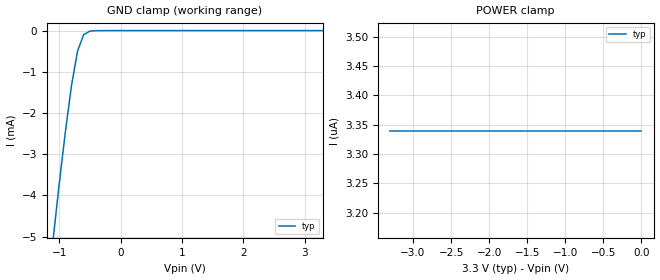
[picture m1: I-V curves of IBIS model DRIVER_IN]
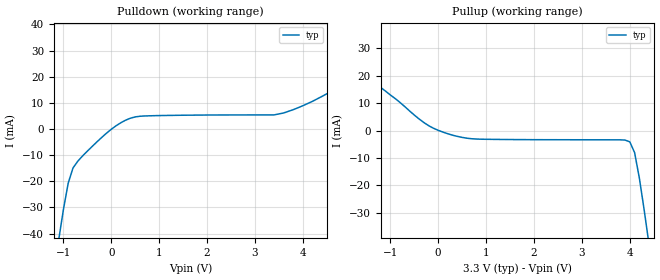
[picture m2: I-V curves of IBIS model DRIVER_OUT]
|   Texas Instruments Incorporated
|   Data Transmissions Products
|   IBIS Model for SN65LVDS1
|   5DBV SOP Package
[IBIS Ver]   2.1
[Comment char]   |_char
[File name]   lvds1.ibs
[File Rev]   1.0
[Date]   11Jan00
[Source]   File originated at Texas Instruments Incorporated.
   Data Transmission Products Group.
[Notes]
[Disclaimer]
(C) Copyright Texas Instruments Incorporated 2000
   All rights reserved
  Texas Instruments Incorporated hereby grants the user of this IBIS
model a non-exclusive, nontransferable license to use this IBIS model
under the following terms.  Before using this IBIS model, the user
should read this license.  If the user does not accept these terms,
the IBIS model should be returned to Texas Instruments within 30 days.
  The user is granted this license only to use the IBIS model and
is not granted rights to sell, load, rent, lease or license the IBIS
model in whole or in part, or in modified form to anyone other than
user.  User may modify the IBIS model to suit its specific applications
but rights to derivative works and such modifications shall belong to
Texas Instruments.
  This IBIS model is provided on an "AS IS" basis and Texas Instruments
makes absolutely no warranty with respect to the information contained
herein.  TEXAS INSTRUMENTS DISCLAIMS AND CUSTOMER WAIVES ALL WARRANTIES,
EXPRESS OR IMPLIED, INCLUDING WARRANTIES OF MERCHANTABILITY OR FITNESS
FOR A PARTICULAR PURPOSE. The entire risk as to quality and performance
is with the Customer. ACCORDINGLY, IN NO EVENT SHALL THE COMPANY BE LIABLE
FOR ANY DAMAGES, WHETHER IN CONTRACT OR TORT,INCLUDING ANY LOST PROFITS
OR OTHER INCIDENTAL, CONSEQUENTIAL, EXEMPLARY, OR PUNITIVE DAMAGES ARISING
OUT OF THE USE OR APPLICATION OF THE IBIS model provided in this package.
Further, Texas Instruments reserves the right to discontinue or make changes
without notice to any product herein to improve reliability, function, or
design. Texas Instruments does not convey any license under patent rights
or any other intellectual property rights, including those of third parties.
Contact Texas Instruments at ATTN:DATA TRANSMISSIONS
[Copyright]   Copyright 2000, Texas Instruments, All Rights Reserved
[Component]   LVDS1DBV
[Manufacturer]  Texas Instruments Incorporated
[Package]
|   typ   min   max
R_pkg   0.036   0.033   0.039
L_pkg   3.340nH   2.445nH   4.233nH
C_pkg   0.470pF   0.308pF   0.631pF
[Pin]   signal_name   model_name   R_pin   L_pin   C_pin
1   VCC   POWER   0.034   4.233n   0.630p
2   GND   GND   0.033   4.231n   0.631p
3   Z   DRIVER_OUT   0.033   4.230n   0.630p
4   Y   DRIVER_OUT   0.033   4.230n   0.630p
5   D   DRIVER_IN   0.033   4.230n   0.630p
[Diff_pin]   inv_pin   vdiff   tdelay_typ   tdelay_min   tdelay_max
| The 'Z' pin is Diff_pin and the 'Y' pin is the inv_pin
4   3   0.100   0 0 0
| Models and submodels in the file (2): DRIVER_IN (Input), DRIVER_OUT (Output)
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|   Driver Input MODEL
[Model]   DRIVER_IN
Model_type   Input
|Signals   D
Vinh = 2.0
Vinl = 0.8
|   typ   min   max
C_comp   1.0pF   NA   NA
|   typ   min   max
[Temperature Range]   25.0   NA   NA
[Voltage range]   3.3V   3.0V   3.6V
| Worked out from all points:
|   GND clamp passes 1 mA (typ) near -0.76 V on its own axis
[GND_clamp]
|   Voltage   I(typ)   I(min)   I(max)
-3.3V     -43.1mA    NA         NA
-1.1V     -5.08mA    NA         NA
-1V       -3.73mA    NA         NA
-900mV    -2.47mA    NA         NA
-800mV    -1.34mA    NA         NA
-700mV    -493uA     NA         NA
-600mV    -98.5uA    NA         NA
-500mV    -13.3uA    NA         NA
3.3V      3.34pA     NA         NA
[Power_clamp]
| Note that the[POWER_clamp]voltage table is referenced to Vcc
| and is calculated using Vtable=Vcc - Vmeasured.
|   Voltage   I(typ)   I(min)   I(max)
-3.3V     3.34uA     NA         NA
-2.7V     3.34uA     NA         NA
-2V       3.34uA     NA         NA
-800mV    3.34uA     NA         NA
0V        3.34uA     NA         NA
[Model]   DRIVER_OUT
Model_type   Output
| Signals   Y,Z
Vmeas = 1.2V   |Reference voltage for timing measurements
Cref = 5pF   |Timing specification test load capacitance value
Rref = 50   |Note: 50 Ohm load; single ended configuration
Vref = 1.18V   |Timing specification test load voltage
| variable   typ   min   max
C_comp   1.0pF   NA   NA
|   typ   min   max
[Temperature Range]   25.0   NA   NA
[Voltage range]   3.3V   3.0V   3.6V
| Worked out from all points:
|   slope of the pulldown table from 0 to 0.495 V, typ, clamps not added: 105 ohm
|   slope of the pullup table from 0 to 0.495 V, typ, clamps not added: 192 ohm
[Pulldown]
|   Voltage   I(typ)   I(min)   I(max)
-3.3V     -348mA     NA         NA
-1.1V     -42.6mA    NA         NA
-900mV    -20.7mA    NA         NA
-800mV    -14.9mA    NA         NA
-300mV    -4.91mA    NA         NA
200mV     2.42mA     NA         NA
600mV     4.89mA     NA         NA
3.4V      5.41mA     NA         NA
3.6V      6.16mA     NA         NA
4.6V      14.5mA     NA         NA
5.6V      26mA       NA         NA
6.6V      38.9mA     NA         NA
[Pullup]
|   Voltage   I(typ)   I(min)   I(max)
| Note that the[Pullup]voltage table is referenced to Vcc
| and is calculated using Vtable=Vcc - Vmeasured.
-3.3V     49.3mA     NA         NA
-2.6V     37.7mA     NA         NA
-1.9V     25.6mA     NA         NA
-400mV    4.24mA     NA         NA
200mV     -1.17mA    NA         NA
800mV     -3.11mA    NA         NA
4V        -4.13mA    NA         NA
4.1V      -8.04mA    NA         NA
4.2V      -17.4mA    NA         NA
4.3V      -29mA      NA         NA
4.4V      -41.4mA    NA         NA
6.6V      -348mA     NA         NA
[Ramp]
|   typ   min   max
dV/dt_r   0.346/600ps   NA   NA
dV/dt_f   0.309/600ps   NA   NA
R_load = 100ohm | Note: The measurement is on a differential configuration
